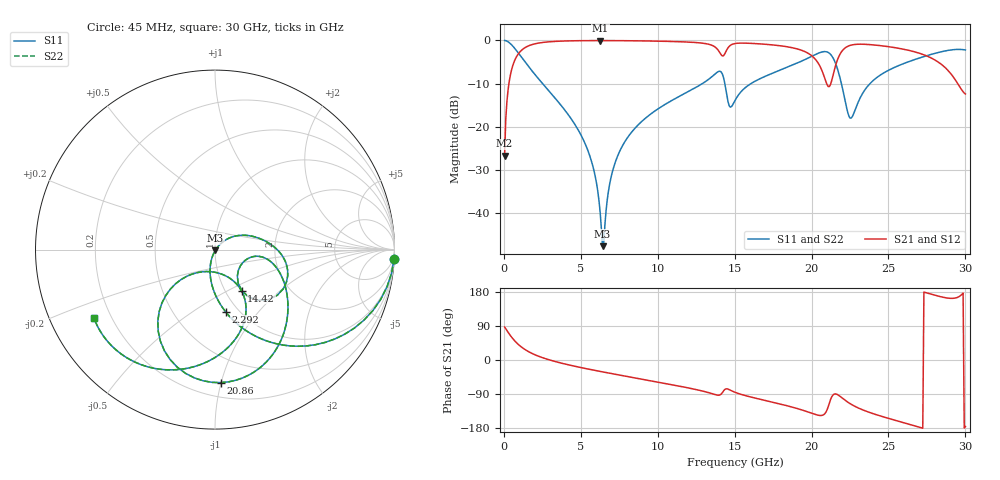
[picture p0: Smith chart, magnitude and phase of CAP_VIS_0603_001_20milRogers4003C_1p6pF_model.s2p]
! S-parameter model data by Modelithics Inc.  support@modelithics.com  813-866-6335  Tampa FL USA
! S-Parameter data specifications:
! Substrate: 20-mil Rogers 4003C, substrate thickness, H=0.508mm, Dielectric constant, Er=3.75
! PCB Mounting Pad Footprint: Pad width, PadW=0.90mm , Pad length, PadL=1.00mm , Pad gap, PadG (edge-to-edge)=1.00mm , Reference planes=3.0mm apart
! Created Wed Nov 18 13:18:46 2015
# hz S ma R 50
! 2 Port Network Data from SP1.SP block
! freq  magS11  angS11  magS21  angS21  magS12  angS12  magS22  angS22
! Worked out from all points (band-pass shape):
!   401 points, 45 MHz to 30 GHz, reference 50 ohm
!   highest |S21| = -0.04 dB at 6.261 GHz (marker M1); lowest = -26.8 dB at 45 MHz (marker M2)
!   |S21| within 3 dB of the highest: 954.5 MHz to 14.07 GHz (13.12 GHz wide, 175 % of centre); 14.37 GHz to 19.8 GHz (5.431 GHz wide, 31.8 % of centre)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
!   lowest |S11| = -47.8 dB at 6.41 GHz (marker M3), VSWR 1.01, Z = 50.2 - j0.334 ohm
!   |S11| at or under -10 dB: 2.509 GHz to 12.91 GHz (10.4 GHz wide, 135 % of centre); 14.36 GHz to 16.07 GHz (1.71 GHz wide, 11.2 % of centre); 21.94 GHz to 23.8 GHz (1.865 GHz wide, 8.16 % of centre)
!   |S22| runs from -47.8 to 0.0 dB; largest |S21 - S12| = 0
!   S11 on the Smith chart (normalised r, x): 45 MHz: 1, -40; 2.292 GHz: 0.87, -0.69; 14.42 GHz: 1.19, -0.59; 20.86 GHz: 0.30, -1.00; 30 GHz: 0.14, -0.26
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4.5e7  0.9989 -2.9  0.04596 87.1  0.04596 87.1  0.9989 -2.9
3.4455e8  0.9428 -21.1  0.333 68.8  0.333 68.8  0.9428 -21.1
6.441e8  0.8325 -36.8  0.5533 53.2  0.5533 53.2  0.8325 -36.8
2.291625e9  0.3513 -80.3  0.934 9.3  0.934 9.3  0.3513 -80.3
5.062462e9  0.07656 -108.0  0.9934 -20.4  0.9934 -20.4  0.07656 -108.0
5.811338e9  0.03312 -110.5  0.9954 -26.6  0.9954 -26.6  0.03312 -110.5
6.260662e9  0.00992 -98.2  0.9957 -30.2  0.9957 -30.2  0.00992 -98.2
6.410438e9  0.004096 -54.2  0.9957 -31.3  0.9957 -31.3  0.004096 -54.2
6.93465e9  0.02437 45.2  0.9951 -35.4  0.9951 -35.4  0.02437 45.2
7.53375e9  0.05206 45.4  0.9938 -39.9  0.9938 -39.9  0.05206 45.4
1.007992e10  0.1633 29.1  0.98 -58.9  0.98 -58.9  0.1633 29.1
1.38243e10  0.4215 -16.2  0.8099 -92.3  0.8099 -92.3  0.4215 -16.2
1.44234e10  0.2724 -56.9  0.7377 -76.3  0.7377 -76.3  0.2724 -56.9
1.50225e10  0.2008 -12.7  0.9198 -85.2  0.9198 -85.2  0.2008 -12.7
1.779334e10  0.44 -27.4  0.8742 -114.5  0.8742 -114.5  0.44 -27.4
2.003996e10  0.6582 -59.6  0.657 -140.9  0.657 -140.9  0.6582 -59.6
2.086372e10  0.7418 -87.5  0.3615 -141.6  0.3615 -141.6  0.7418 -87.5
2.16126e10  0.5103 -128.6  0.5469 -90.0  0.5469 -90.0  0.5103 -128.6
2.251125e10  0.1253 -100.8  0.8759 -115.3  0.8759 -115.3  0.1253 -100.8
2.505742e10  0.4556 -70.4  0.8433 -154.7  0.8433 -154.7  0.4556 -70.4
2.812781e10  0.7159 -110.6  0.5769 169.8  0.5769 169.8  0.7159 -110.6
3e10  0.7749 -150.4  0.2391 -175.4  0.2391 -175.4  0.7749 -150.4
